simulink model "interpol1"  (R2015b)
settings: Solver=VariableStepAuto  StartTime=0.0  StopTime=10.0  RelTol=1e-3
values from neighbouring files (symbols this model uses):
  a = 1/(Tsig/2.5)    (= 7.8125)    [fourier_transf_puls_3.m]    (also in fourier_transf_puls_4.m; schar_1.m = 5)
  b = 10    [schar_1.m]
  hint = fir1(nord, 0.9*1/L)    [interpol_1.m]    (also in interpol_2.m = fir1(nord, 1/L); poly_interp_1.m = fir1(nord2, 1/L); poly_interp_2.m = fir1(nord2, 1/L))
  L = 3    [farrow_3.m]    (also in farrow_4.m = 480; ifir_1.m = 5; ifir_dezim_1.m = 5; ifir_high1.m = 5)
  nord = 6    [dezimier_1.m]    (also in dezimier_11.m; dezimier_2.m = 256; dezimier_3.m = 256; farrow_2.m = 128)
  Ts = 1/fs    (= 5e-05)    [basisband_1.m]    (also in basisband_2.m = 5e-06; dezimier_1.m = 0.0005; dezimier_11.m = 0.0005; dezimier_2.m = 0.0005)
libraries: dspsigops x1

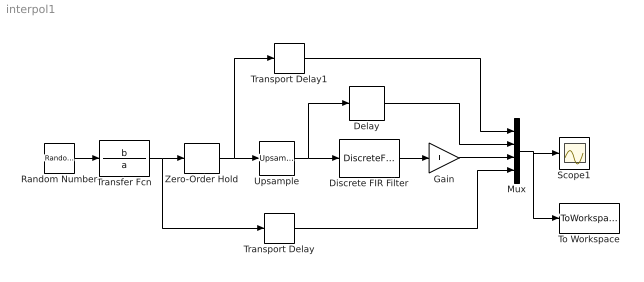
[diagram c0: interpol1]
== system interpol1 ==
  Delay : Delay  DelayLength=nord/2
  Discrete FIR Filter : DiscreteFir  Coefficients=hint  SampleTime=Ts/L
  Gain : Gain  Gain=L
  Mux : Mux
  Random Number : RandomNumber  Seed=03678  SampleTime=0
  Scope1 : Scope
  To Workspace : ToWorkspace  VariableName=y  SaveFormat=Timeseries  SampleTime=-1
  Transfer Fcn : TransferFcn  Numerator=b  Denominator=a
  Transport Delay : TransportDelay  DelayTime=nord*Ts/(2*L)  BufferSize=1024*2
  Transport Delay1 : TransportDelay  DelayTime=nord*Ts/(2*L)  BufferSize=1024*2
  Upsample : dspsigops/Upsample  N=L  phase=0  RateOptions=Allow multirate processing  ic=0  mode=Unused parameter value
  Zero-Order Hold : ZeroOrderHold  SampleTime=Ts
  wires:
  Random Number/1 -> Transfer Fcn/1
  Upsample/1 -> Delay/1, Discrete FIR Filter/1
  Discrete FIR Filter/1 -> Gain/1
  Delay/1 -> Mux/2
  Gain/1 -> Mux/3
  Transfer Fcn/1 -> Transport Delay/1, Zero-Order Hold/1
  Mux/1 -> To Workspace/1, Scope1/1
  Transport Delay/1 -> Mux/4
  Zero-Order Hold/1 -> Transport Delay1/1, Upsample/1
  Transport Delay1/1 -> Mux/1
